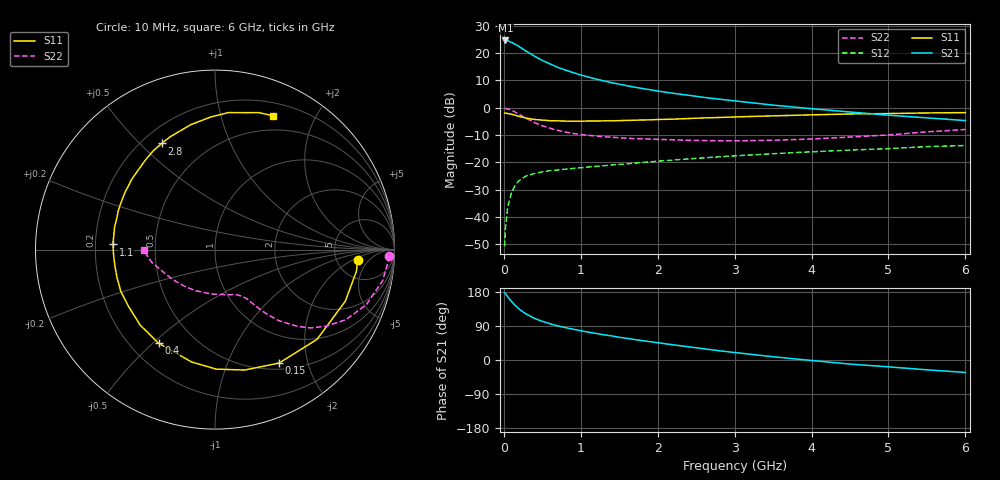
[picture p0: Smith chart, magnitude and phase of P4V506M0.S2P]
! SIEMENS Small Signal Semiconductors
! BFP182
! Si NPN RF Bipolar Junction Transistor in SOT143
! VCE = 0.5 V  IC = 6 mA
! Common Emitter S-Parameters:  March  1996
# GHz  S  MA  R  50
!  f  S11  S21  S12  S22
! GHz  MAG  ANG  MAG  ANG  MAG  ANG  MAG  ANG
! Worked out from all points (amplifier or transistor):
!   36 points, 10 MHz to 6 GHz, reference 50 ohm
!   highest |S21| = 24.6 dB at 20 MHz (marker M1)
!   |S21| within 3 dB of that: start of sweep to 238.9 MHz
!   unconditionally stable (mu >= 1): 1.101 GHz to end of sweep
!   at 250 MHz: K = 0.29, MSG = 23.6 dB, |S12| = -25.7 dB
!   at 1.4 GHz: K = 1.16, MAG = 12.7 dB, |S12| = -21.0 dB
!   at 6 GHz: K = 1.24, MAG = 1.6 dB, |S12| = -13.9 dB
!   S11 on the Smith chart (normalised r, x): 10 MHz: 7.98, -2.61; 150 MHz: 0.58, -1.56; 400 MHz: 0.31, -0.52; 1.1 GHz: 0.27, +0.02; 2.8 GHz: 0.28, +0.58; 6 GHz: 0.33, +1.47
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0.01  0.7968 -4.3  16.91 177.6  0.0029 86.8  0.9681 -2.1
0.02  0.7972 -8.7  17.06 175.2  0.006 80.5  0.9668 -4.2
0.05  0.781 -21.6  16.83 166.7  0.0151 79.9  0.9494 -10.6
0.1  0.7571 -41.3  15.69 154.5  0.0278 68.6  0.8964 -20.1
0.15  0.7261 -60.5  14.48 143.5  0.0386 59.8  0.8266 -28.2
0.2  0.6913 -76.1  13.16 134.3  0.0463 53.8  0.7533 -34.5
0.25  0.6659 -89.4  11.78 126.7  0.0519 47.7  0.6877 -39.4
0.3  0.6397 -101.7  10.68 120.4  0.0569 44.1  0.6286 -42.9
0.4  0.6089 -121.0  8.768 109.6  0.0623 38.2  0.5319 -48.1
0.5  0.5923 -134.7  7.331 102.0  0.0667 34.5  0.4655 -51.0
0.6  0.5767 -146.5  6.336 95.6  0.0704 32.5  0.4202 -52.9
0.7  0.5743 -156.0  5.488 90.2  0.072 31.2  0.3841 -54.2
0.9  0.5652 -170.7  4.392 81.3  0.0771 30.0  0.3372 -56.3
1.1  0.5695 177.1  3.644 73.4  0.082 29.6  0.3117 -58.6
1.5  0.5801 158.6  2.693 60.0  0.0912 29.5  0.2814 -63.8
1.8  0.5955 146.8  2.253 51.1  0.0991 29.6  0.2691 -68.9
2.2  0.6164 133.8  1.837 40.1  0.1098 28.5  0.2574 -77.5
2.8  0.6616 116.6  1.432 24.4  0.1258 25.9  0.2482 -93.1
3.5  0.7089 101.0  1.115 8.6  0.1435 21.8  0.253 -114.9
4.5  0.7674 84.3  0.833 -10.7  0.1672 15.1  0.2895 -145.0
5.5  0.8012 72.3  0.651 -25.9  0.1933 8.4  0.361 -169.0
6  0.8121 66.7  0.581 -32.8  0.2029 3.9  0.3982 -179.6
